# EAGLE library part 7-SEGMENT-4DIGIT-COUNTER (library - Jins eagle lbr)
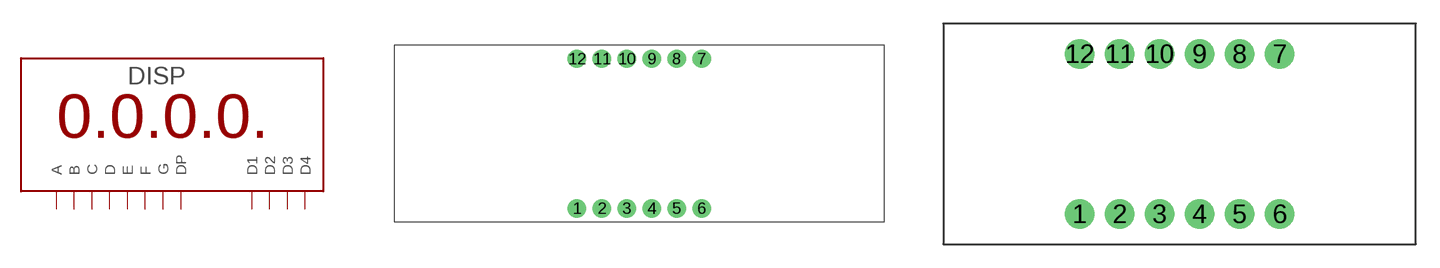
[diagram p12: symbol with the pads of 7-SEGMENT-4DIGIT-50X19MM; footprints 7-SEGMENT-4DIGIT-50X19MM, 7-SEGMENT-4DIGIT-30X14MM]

Designator prefix DISP

## 7-SEGMENT-4DIGIT-COUNTERPTH  [7-SEGMENT-4DIGIT-50X19MM]
1  E
2  D
3  DP
4  C
5  G
6  D4
7  B
8  D3
9  D2
10  F
11  A
12  D1

## 7-SEGMENT-4DIGIT-COUNTERPTH-S  [7-SEGMENT-4DIGIT-30X14MM]
Pads as for 7-SEGMENT-4DIGIT-50X19MM

## Footprint 7-SEGMENT-4DIGIT-50X19MM (pad centres in mm)
drill 0.9 pad 1.88: 1 -6.35,-7.62; 2 -3.81,-7.62; 3 -1.27,-7.62; 4 1.27,-7.62; 5 3.81,-7.62; 6 6.35,-7.62; 7 6.35,7.62; 8 3.81,7.62; 9 1.27,7.62; 10 -1.27,7.62; 11 -3.81,7.62; 12 -6.35,7.62

## Footprint 7-SEGMENT-4DIGIT-30X14MM (pad centres in mm)
drill 0.9 pad 1.88: 1 -6.35,-5.08; 2 -3.81,-5.08; 3 -1.27,-5.08; 4 1.27,-5.08; 5 3.81,-5.08; 6 6.35,-5.08; 7 6.35,5.08; 8 3.81,5.08; 9 1.27,5.08; 10 -1.27,5.08; 11 -3.81,5.08; 12 -6.35,5.08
